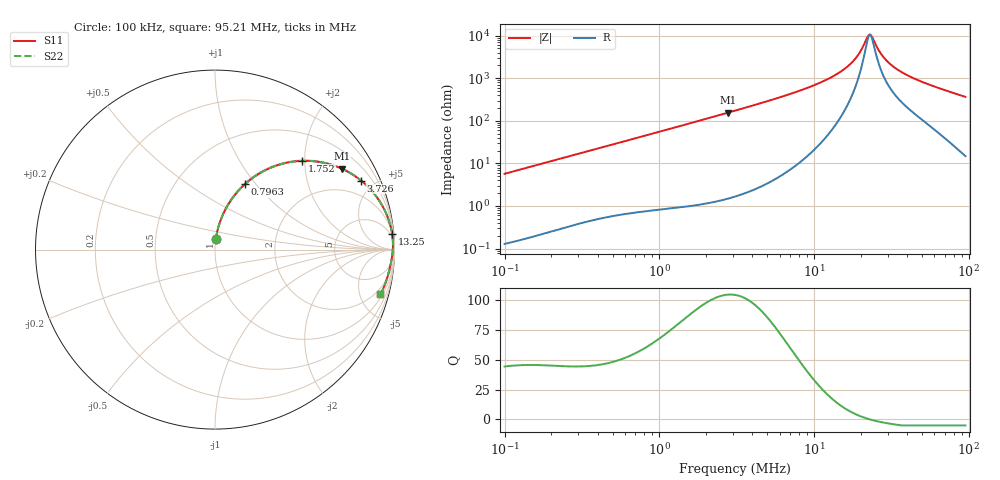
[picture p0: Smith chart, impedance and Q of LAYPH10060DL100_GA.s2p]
! LAYPH10060DL100_GA  S-PARAMETER MODEL  ( General Type )
! Model Generated by TAIYO YUDEN Corporation (http://www.ty-top.com)
! Version 3.0
! TAIYO YUDEN Control No. 180828NI43SB-FBB
! Copyright(c) 2017 TAIYO YUDEN CO.,LTD. All Rights Reserved.
! Product Description (link to TY-COMPAS)
! https://ds.yuden.co.jp/TYCOMPAS/or/detail?pn=LAYPH10060DL100MGA&u=M
! Products Name : Inductors
! Characteristics :
!  Inductance : 10 uH , SRF(min) : -Hz , DC Resistance(max) : 0.026 Ohm
!  Rated Current : Saturation :4.3 A , Temp Rise : 3 A (25 degC)
!  Case Size : 10.1 x 10.0 / 0.398 x 0.394 [mm/inch] , Thickness : 6 / 0.236 [mm/inch]
!  (Conditions: Temperature = 25 degC , DC Bias Current/Voltage = 0A / 0V)
! External Node Assignments :
!  1  o---GGG---o  2
! GND o---------o GND
! Frequency Range : 0.1MHz  -  95.211795MHz  [ 402 STEP ]
# MHz S RI R 50
! Freq[MHz].  S11 Real  S11 Imag  S21 Real  S21 Imag  S12 Real  S12 Imag  S22 Real  S22 Imag
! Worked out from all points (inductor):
!   401 points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, 100 kHz to 95.21 MHz, reference 50 ohm
!   read as one part in series: L = 9.06 uH near 103.5 kHz
!   highest Q = 104 at 2.784 MHz (marker M1), where L = 8.9 uH
!   self-resonance near 22.94 MHz
!   S11 on the Smith chart (normalised r, x): 100 kHz: 1.00, +0.11; 796.3 kHz: 1.01, +0.88; 1.752 MHz: 1.02, +1.94; 3.726 MHz: 1.04, +4.22; 13.25 MHz: 2, +22; 95.21 MHz: 1.30, -7.30
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0.1  0.00452 0.0568  0.9955 -0.0568  0.9955 -0.0568  0.00452 0.0568
0.31545  0.0341 0.1707  0.9659 -0.1707  0.9659 -0.1707  0.0341 0.1707
0.796258  0.1675 0.3651  0.8325 -0.3651  0.8325 -0.3651  0.1675 0.3651
0.995088  0.2365 0.4176  0.7635 -0.4176  0.7635 -0.4176  0.2365 0.4176
1.75228  0.486 0.4944  0.514 -0.4944  0.514 -0.4944  0.486 0.4944
2.783973  0.7063 0.4507  0.2937 -0.4507  0.2937 -0.4507  0.7063 0.4507
3.085641  0.748 0.4294  0.252 -0.4294  0.252 -0.4294  0.748 0.4294
3.726142  0.8142 0.384  0.1858 -0.384  0.1858 -0.384  0.8142 0.384
5.720415  0.916 0.2709  0.084 -0.2709  0.084 -0.2709  0.916 0.2709
9.733658  0.9734 0.1472  0.0266 -0.1472  0.0266 -0.1472  0.9734 0.1472
13.25309  0.9867 0.0885  0.0133 -0.0885  0.0133 -0.0885  0.9867 0.0885
15.73202  0.9902 0.0593  0.00983 -0.0593  0.00983 -0.0593  0.9902 0.0593
18.04506  0.9914 0.0372  0.00861 -0.0372  0.00861 -0.0372  0.9914 0.0372
20.0004  0.9915 0.0213  0.00848 -0.0213  0.00848 -0.0213  0.9915 0.0213
22.16762  0.991 0.00575  0.00897 -0.00575  0.00897 -0.00575  0.991 0.00575
22.941  0.9907 0.000659  0.00926 -0.000659  0.00926 -0.000659  0.9907 0.000659
23.74138  0.9904 -0.0044  0.00962 0.0044  0.00962 0.0044  0.9904 -0.0044
27.23201  0.9884 -0.0244  0.0116 0.0244  0.0116 0.0244  0.9884 -0.0244
30.70484  0.986 -0.0417  0.014 0.0417  0.014 0.0417  0.986 -0.0417
36.44803  0.9816 -0.0666  0.0184 0.0666  0.0184 0.0666  0.9816 -0.0666
45.54928  0.9744 -0.1004  0.0256 0.1004  0.0256 0.1004  0.9744 -0.1004
95.21179  0.9216 -0.2492  0.0784 0.2492  0.0784 0.2492  0.9216 -0.2492
